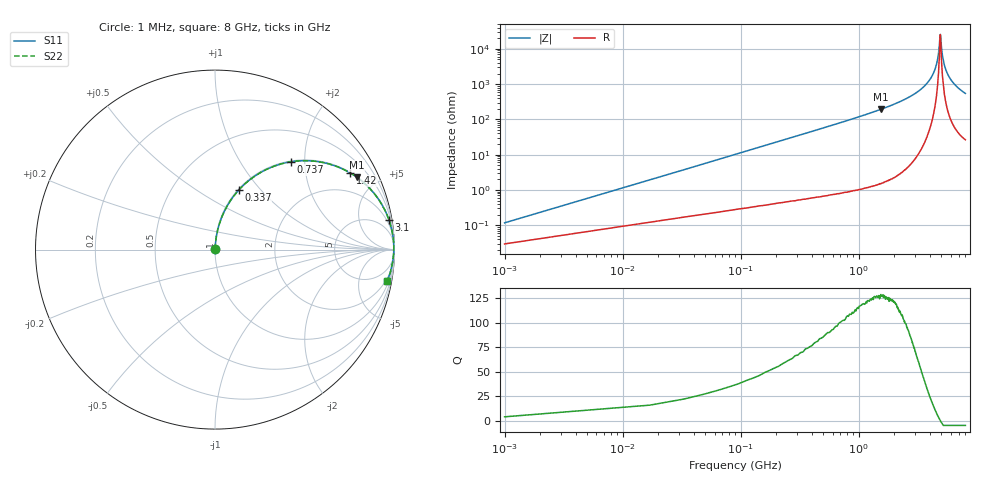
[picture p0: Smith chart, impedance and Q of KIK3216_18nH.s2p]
!version-2
!date-01.2022
!Series
# MHz S RI R 50
!Freq ReS11 ImS11 ReS21 ImS21 ReS12 ImS12 ReS22 ImS22
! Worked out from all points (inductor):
!   501 points, 1 MHz to 8 GHz, reference 50 ohm
!   read as one part in series: L = 18 nH near 33 MHz
!   highest Q = 128 at 1.55 GHz (marker M1), where L = 20 nH
!   self-resonance near 4.9 GHz
!   S11 on the Smith chart (normalised r, x): 1 MHz: 1.00, +0.00; 337 MHz: 1.01, +0.77; 737 MHz: 1.02, +1.71; 1.42 GHz: 1.03, +3.52; 3.1 GHz: 1, +12; 8 GHz: 2, -11
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1  0.000292 0.00113  0.9997 -0.00113  0.9997 -0.00113  0.000292 0.00113
49  0.00508 0.055  0.9949 -0.055  0.9949 -0.055  0.00508 0.055
81  0.0109 0.0904  0.9891 -0.0904  0.9891 -0.0904  0.0109 0.0904
177  0.0421 0.1913  0.9579 -0.1913  0.9579 -0.1913  0.0421 0.1913
337  0.1314 0.3308  0.8686 -0.3308  0.8686 -0.3308  0.1314 0.3308
737  0.4218 0.489  0.5782 -0.489  0.5782 -0.489  0.4218 0.489
1340  0.7285 0.4408  0.2715 -0.4408  0.2715 -0.4408  0.7285 0.4408
1420  0.7543 0.4266  0.2457 -0.4266  0.2457 -0.4266  0.7543 0.4266
1550  0.7903 0.4032  0.2097 -0.4032  0.2097 -0.4032  0.7903 0.4032
2670  0.9465 0.2196  0.0535 -0.2196  0.0535 -0.2196  0.9465 0.2196
3100  0.9693 0.1651  0.0307 -0.1651  0.0307 -0.1651  0.9693 0.1651
4020  0.9918 0.0718  0.00824 -0.0718  0.00824 -0.0718  0.9918 0.0718
4310  0.9945 0.0469  0.00549 -0.0469  0.00549 -0.0469  0.9945 0.0469
4580  0.9959 0.0249  0.00415 -0.0249  0.00415 -0.0249  0.9959 0.0249
4740  0.9962 0.0126  0.00385 -0.0126  0.00385 -0.0126  0.9962 0.0126
4900  0.9961 0.000756  0.00386 -0.000756  0.00386 -0.000756  0.9961 0.000756
4930  0.9961 -0.00157  0.0039 0.00157  0.0039 0.00157  0.9961 -0.00157
5100  0.9957 -0.0141  0.00429 0.0141  0.00429 0.0141  0.9957 -0.0141
5350  0.9947 -0.0305  0.00532 0.0305  0.00532 0.0305  0.9947 -0.0305
5820  0.9912 -0.0612  0.0088 0.0612  0.0088 0.0612  0.9912 -0.0612
6670  0.9814 -0.1096  0.0186 0.1096  0.0186 0.1096  0.9814 -0.1096
8000  0.9596 -0.1741  0.0404 0.1741  0.0404 0.1741  0.9596 -0.1741
